| IBIS file stm32f413_f423_wlcsp100.ibs
[IBIS ver] 4.2
[File name] stm32f413_f423_wlcsp100.ibs
[File Rev] 1.2
[Date]  18-05-2020
[Source] Data Created at STMicroelectronics
[Notes]  File originated from ELDO simulations. rev 1.1: removal of the rising/falling waveform I2C
[Disclaimer]  This information is for modeling purpose only and is
   not guaranted. The information is subject to change without
   notice.
[Copyright] Copyright 2020 STMicroelectronics Inc.
|   Component stm32f413_f423_wlcsp100
[Component] stm32f413_f423_wlcsp100
[Manufacturer] STMicroelectronics
[Package]
| variable   typ   min   max
R_pkg   0.0   0.0   0.0
L_pkg   0.0H   0.0H   0.0H
C_pkg   0.0F   0.0F   0.0F
[Pin]  signal_name   model_name   R_pin   L_pin   C_pin
1 PA14 io8p_arsudq_ft
A10 PE4 io8p_arsudq_ft
A2 PC12 io8p_arsudq_ft
A3 PD2 io8p_arsudq_ft
A4 PD5 io8p_arsudq_ft
A5 PD7 io8p_arsudq_ft
A6 PB5 io8p_ar3wsudq_ft
A7 PB8 io8p_arsudq_i2cin_ft
A8 VSS_3 GND
A9 VDD_3 POWER
B1 VDD_2_0 POWER
B10 VBAT POWER
B2 VSS_2_0 GND
B3 PC11 io8p_arsudq_ft
B4 PD1 io8p_arsudq_ft
B5 PD3 io8p_arsudq_ft
B6 PD6 io8p_arsudq_ft
B7 PB6 io8p_arsudq_i2cin_ft
B8 PE0 io8p_arsudq_ft
B9 PE2 io8p_arsudq_ft
C1 VCAP2_0 POWER
C10 PC13-ANTI_TAMP io8p_arwsudq_ft_v33
C2 PA15 io8p_arsudq_ft
C3 PA13 io8p_arsudq_ft
C4 PA10 io8usb_id_otg_ft
C5 PD0 io8p_arsudq_ft
C6 PD4 io8p_arsudq_ft
C7 PB4 io8p_arsudq_i2cin_ft
C8 PE1 io8p_arsudq_ft
C9 PE3 io8p_arsudq_ft
D1 PA11 io8usb_lsfs_otg_ft
D10 PC14-OSC32_IN io8p_arwsudq_ft
D2 PA12 io8usb_lsfs_otg_ft
D3 PA9 io8usb_vbus_otg_ft
D4 PA8 io8p_arsudq_i2cin_ft
D5 PD14 io8p_arsudq_i2c_ft
D6 PB3 io8p_arsudq_i2c_ft
D7 PB7 io8p_arsudq_i2cin_ft
D8 VSS GND
D9 PE5 io8p_arsudq_ft
E1 PC9 io8p_arsudq_i2cin_ft
E10 VSS_5 GND
E2 PC8 io8p_arsudq_ft
E3 PC7 io8p_arsudq_i2c_ft
E4 PB12 io8p_arsudq_ft
E5 PA4 io8p_ar3wsudq_ft
E6 BOOT0 vpp_test_hv
E7 PB9 io8p_arsudq_i2cin_ft
E8 PE6 io8p_arsudq_ft
E9 PC15-OSC32_OUT io8p_arsudq_ft
F1 PC6 io8p_arsudq_i2c_ft
F10 VDD_5 POWER
F2 VDD_2_USB33 POWER
F3 PD10 io8p_arsudq_ft
F4 PE11 io8p_arsudq_ft
F5 PA5 io8p_ar3wsudq_ft
F6 PC3 io8p_arwsudq_ft
F7 PC0 io8p_arwsudq_ft_v33
F8 NRST ioreset_ft_v33
F9 PH0-OSC_IN io8p_arsudq_ft
G1 PD15 io8p_arsudq_i2c_ft
G10 PH1-OSC_OUT io8p_arsudq_ft
G2 PD13 io8p_arsudq_i2c_ft
G3 PD9 io8p_arsudq_ft
G4 PE15 io8p_ar3wsudq_ft
G5 PB2 io8p_arwsudq_ft
G6 PC5 io8p_arwsudq_ft
G7 PA3 io8p_arwsudq_ft
G8 VDDA POWER
G9 PC2 io8p_arwsudq_ft
H1 PD12 io8p_arsudq_i2c_ft
H10 PC1 io8p_arwsudq_ft_v33
H2 PB13 io8p_arsudq_ft
H3 PB10 io8p_arsudq_i2c_ft
H4 PE13 io8p_arsudq_ft
H5 PE7 io8p_arsudq_ft
H6 PC4 io8p_arwsudq_ft
H7 VSS_4 GND
H8 PA0-WKUP io8p_arwsudq_ft_v33
H9 VSSA GND
J1 PD11 io8p_arsudq_ft
J10 VREF+ POWER
J2 PB14 io8p_arsudq_i2c_ft
J3 VCAP1_0 POWER
J4 PE12 io8p_arsudq_ft
J5 PE9 io8p_arsudq_ft
J6 PB1 io8p_ar3wsudq_ft
J7 PA7 io8p_arwsudq_ft
J8 VDD_4 POWER
J9 PA2 io8p_arwsudq_ft
K1 PB15 io8p_arsudq_i2c_ft
K10 PA1 io8p_arwsudq_ft
K2 VDD_1_0 POWER
K3 VSS_1_0 GND
K4 PE14 io8p_arsudq_ft
K5 PE10 io8p_arsudq_ft
K6 PE8 io8p_arsudq_ft
K7 PB0 io8p_ar3wsudq_ft
K8 PA6 io8p_ar3wsudq_ft
K9 BYPASS_USER GND
[Model Selector] io8p_ar3wsudq_ft
io8p00_ar3wsudq_ft_pd_lv  "SPEED00 1P8V, PD=40kOhm"
io8p00_ar3wsudq_ft_pu_lv  "SPEED00 1P8V, PU=40kOhm"
io8p00_ar3wsudq_ft_lv  "SPEED00 1P8V"
io8p01_ar3wsudq_ft_pd_lv  "SPEED01 1P8V, PD=40kOhm"
io8p01_ar3wsudq_ft_pu_lv  "SPEED01 1P8V, PU=40kOhm"
io8p01_ar3wsudq_ft_lv  "SPEED01 1P8V"
io8p10_ar3wsudq_ft_pd_lv  "SPEED10 1P8V, PD=40kOhm"
io8p10_ar3wsudq_ft_pu_lv  "SPEED10 1P8V, PU=40kOhm"
io8p10_ar3wsudq_ft_lv  "SPEED10 1P8V"
io8p11_ar3wsudq_ft_pd_lv  "SPEED11 1P8V, PD=40kOhm"
io8p11_ar3wsudq_ft_pu_lv  "SPEED11 1P8V, PU=40kOhm"
io8p11_ar3wsudq_ft_lv  "SPEED11 1P8V"
io8p00_ar3wsudq_ft_pd  "SPEED00, PD=40kOhm"
io8p00_ar3wsudq_ft_pu  "SPEED00, PU=40kOhm"
io8p00_ar3wsudq_ft  "SPEED00"
io8p01_ar3wsudq_ft_pd  "SPEED01, PD=40kOhm"
io8p01_ar3wsudq_ft_pu  "SPEED01, PU=40kOhm"
io8p01_ar3wsudq_ft  "SPEED01"
io8p10_ar3wsudq_ft_pd  "SPEED10, PD=40kOhm"
io8p10_ar3wsudq_ft_pu  "SPEED10, PU=40kOhm"
io8p10_ar3wsudq_ft  "SPEED10"
io8p11_ar3wsudq_ft_pd  "SPEED11, PD=40kOhm"
io8p11_ar3wsudq_ft_pu  "SPEED11, PU=40kOhm"
io8p11_ar3wsudq_ft  "SPEED11"
[Model Selector] io8p_arsudq_ft
io8p00_arsudq_ft_pd_lv  "SPEED00 1P8V, PD=40kOhm"
io8p00_arsudq_ft_pu_lv  "SPEED00 1P8V, PU=40kOhm"
io8p00_arsudq_ft_lv  "SPEED00 1P8V"
io8p01_arsudq_ft_pd_lv  "SPEED01 1P8V, PD=40kOhm"
io8p01_arsudq_ft_pu_lv  "SPEED01 1P8V, PU=40kOhm"
io8p01_arsudq_ft_lv  "SPEED01 1P8V"
io8p10_arsudq_ft_pd_lv  "SPEED10 1P8V, PD=40kOhm"
io8p10_arsudq_ft_pu_lv  "SPEED10 1P8V, PU=40kOhm"
io8p10_arsudq_ft_lv  "SPEED10 1P8V"
io8p11_arsudq_ft_pd_lv  "SPEED11 1P8V, PD=40kOhm"
io8p11_arsudq_ft_pu_lv  "SPEED11 1P8V, PU=40kOhm"
io8p11_arsudq_ft_lv  "SPEED11 1P8V"
io8p00_arsudq_ft_pd  "SPEED00, PD=40kOhm"
io8p00_arsudq_ft_pu  "SPEED00, PU=40kOhm"
io8p00_arsudq_ft  "SPEED00"
io8p01_arsudq_ft_pd  "SPEED01, PD=40kOhm"
io8p01_arsudq_ft_pu  "SPEED01, PU=40kOhm"
io8p01_arsudq_ft  "SPEED01"
io8p10_arsudq_ft_pd  "SPEED10, PD=40kOhm"
io8p10_arsudq_ft_pu  "SPEED10, PU=40kOhm"
io8p10_arsudq_ft  "SPEED10"
io8p11_arsudq_ft_pd  "SPEED11, PD=40kOhm"
io8p11_arsudq_ft_pu  "SPEED11, PU=40kOhm"
io8p11_arsudq_ft  "SPEED11"
[Model Selector] io8p_arsudq_i2c_ft
io8prog_1v8_i2c_pd  "5V Tol GPIO 1.8V range i2c functionality with pull down"
io8prog_1v8_i2c_pu  "5V Tol GPIO 1.8V range i2c functionality with pull up"
io8prog_1v8_i2c  "5V Tol GPIO 1.8V range i2c functionality"
io8prog_3v3_i2c_pd  "5V Tol GPIO 3.3V range i2c functionality with pull down"
io8prog_3v3_i2c_pu  "5V Tol GPIO 3.3V range i2c functionality with pull up"
io8prog_3v3_i2c  "5V Tol GPIO 3.3V range i2c functionality"
io8prog_1v8_pd_00  "5V Tol GPIO 1.8V range with pd speed 00"
io8prog_1v8_pu_00  "5V Tol GPIO 1.8V range with pu speed 00"
io8prog_1v8_00  "5V Tol GPIO 1.8V range speed 00"
io8prog_3v3_pd_00  "5V Tol GPIO 3.3V range with pd speed 00"
io8prog_3v3_pu_00  "5V Tol GPIO 3.3V range with pu speed 00"
io8prog_3v3_00  "5V Tol GPIO 3.3V range speed 00"
io8prog_1v8_pd_01  "5V Tol GPIO 1.8V range with pd speed 01"
io8prog_1v8_pu_01  "5V Tol GPIO 1.8V range with pu speed 01"
io8prog_1v8_01  "5V Tol GPIO 1.8V range speed 01"
io8prog_3v3_pd_01  "5V Tol GPIO 3.3V range with pd speed 01"
io8prog_3v3_pu_01  "5V Tol GPIO 3.3V range with pu speed 01"
io8prog_3v3_01  "5V Tol GPIO 3.3V range speed 01"
io8prog_1v8_pd_10  "5V Tol GPIO 1.8V range with pd speed 10"
io8prog_1v8_pu_10  "5V Tol GPIO 1.8V range with pu speed 10"
io8prog_1v8_10  "5V Tol GPIO 1.8V range speed 10"
io8prog_3v3_pd_10  "5V Tol GPIO 3.3V range with pd speed 10"
io8prog_3v3_pu_10  "5V Tol GPIO 3.3V range with pu speed 10"
io8prog_3v3_10  "5V Tol GPIO 3.3V range speed 10"
io8prog_1v8_pd_11  "5V Tol GPIO 1.8V range with pd speed 11"
io8prog_1v8_pu_11  "5V Tol GPIO 1.8V range with pu speed 11"
io8prog_1v8_11  "5V Tol GPIO 1.8V range speed 11"
io8prog_3v3_pd_11  "5V Tol GPIO 3.3V range with pd speed 11"
io8prog_3v3_pu_11  "5V Tol GPIO 3.3V range with pu speed 11"
io8prog_3v3_11  "5V Tol GPIO 3.3V range speed 11"
[Model Selector] io8p_arsudq_i2cin_ft
io8p00_arsudq_i2cin_ft_pd_lv  "SPEED00 1P8V, PD=40kOhm"
io8p00_arsudq_i2cin_ft_pu_lv  "SPEED00 1P8V, PU=40kOhm"
io8p00_arsudq_i2cin_ft_lv  "SPEED00 1P8V"
io8p01_arsudq_i2cin_ft_pd_lv  "SPEED01 1P8V, PD=40kOhm"
io8p01_arsudq_i2cin_ft_pu_lv  "SPEED01 1P8V, PU=40kOhm"
io8p01_arsudq_i2cin_ft_lv  "SPEED01 1P8V"
io8p10_arsudq_i2cin_ft_pd_lv  "SPEED10 1P8V, PD=40kOhm"
io8p10_arsudq_i2cin_ft_pu_lv  "SPEED10 1P8V, PU=40kOhm"
io8p10_arsudq_i2cin_ft_lv  "SPEED10 1P8V"
io8p11_arsudq_i2cin_ft_pd_lv  "SPEED11 1P8V, PD=40kOhm"
io8p11_arsudq_i2cin_ft_pu_lv  "SPEED11 1P8V, PU=40kOhm"
io8p11_arsudq_i2cin_ft_lv  "SPEED11 1P8V"
io8p00_arsudq_i2cin_ft_pd  "SPEED00, PD=40kOhm"
io8p00_arsudq_i2cin_ft_pu  "SPEED00, PU=40kOhm"
io8p00_arsudq_i2cin_ft  "SPEED00"
io8p01_arsudq_i2cin_ft_pd  "SPEED01, PD=40kOhm"
io8p01_arsudq_i2cin_ft_pu  "SPEED01, PU=40kOhm"
io8p01_arsudq_i2cin_ft  "SPEED01"
io8p10_arsudq_i2cin_ft_pd  "SPEED10, PD=40kOhm"
io8p10_arsudq_i2cin_ft_pu  "SPEED10, PU=40kOhm"
io8p10_arsudq_i2cin_ft  "SPEED10"
io8p11_arsudq_i2cin_ft_pd  "SPEED11, PD=40kOhm"
io8p11_arsudq_i2cin_ft_pu  "SPEED11, PU=40kOhm"
io8p11_arsudq_i2cin_ft  "SPEED11"
[Model Selector] io8p_arwsudq_ft
io8p00_arwsudq_ft_pd_lv  "SPEED00 1P8V, PD=40kOhm"
io8p00_arwsudq_ft_pu_lv  "SPEED00 1P8V, PU=40kOhm"
io8p00_arwsudq_ft_lv  "SPEED00 1P8V"
io8p01_arwsudq_ft_pd_lv  "SPEED01 1P8V, PD=40kOhm"
io8p01_arwsudq_ft_pu_lv  "SPEED01 1P8V, PU=40kOhm"
io8p01_arwsudq_ft_lv  "SPEED01 1P8V"
io8p10_arwsudq_ft_pd_lv  "SPEED10 1P8V, PD=40kOhm"
io8p10_arwsudq_ft_pu_lv  "SPEED10 1P8V, PU=40kOhm"
io8p10_arwsudq_ft_lv  "SPEED10 1P8V"
io8p11_arwsudq_ft_pd_lv  "SPEED11 1P8V, PD=40kOhm"
io8p11_arwsudq_ft_pu_lv  "SPEED11 1P8V, PU=40kOhm"
io8p11_arwsudq_ft_lv  "SPEED11 1P8V"
io8p00_arwsudq_ft_pd  "SPEED00, PD=40kOhm"
io8p00_arwsudq_ft_pu  "SPEED00, PU=40kOhm"
io8p00_arwsudq_ft  "SPEED00"
io8p01_arwsudq_ft_pd  "SPEED01, PD=40kOhm"
io8p01_arwsudq_ft_pu  "SPEED01, PU=40kOhm"
io8p01_arwsudq_ft  "SPEED01"
io8p10_arwsudq_ft_pd  "SPEED10, PD=40kOhm"
io8p10_arwsudq_ft_pu  "SPEED10, PU=40kOhm"
io8p10_arwsudq_ft  "SPEED10"
io8p11_arwsudq_ft_pd  "SPEED11, PD=40kOhm"
io8p11_arwsudq_ft_pu  "SPEED11, PU=40kOhm"
io8p11_arwsudq_ft  "SPEED11"
[Model Selector] io8p_arwsudq_ft_v33
io8p00_arwsudq_ft_v33_pd_lv  "SPEED00 1P8V, PD=40kOhm"
io8p00_arwsudq_ft_v33_pu_lv  "SPEED00 1P8V, PU=40kOhm"
io8p00_arwsudq_ft_v33_lv  "SPEED00 1P8V"
io8p01_arwsudq_ft_v33_pd_lv  "SPEED01 1P8V, PD=40kOhm"
io8p01_arwsudq_ft_v33_pu_lv  "SPEED01 1P8V, PU=40kOhm"
io8p01_arwsudq_ft_v33_lv  "SPEED01 1P8V"
io8p10_arwsudq_ft_v33_pd_lv  "SPEED10 1P8V, PD=40kOhm"
io8p10_arwsudq_ft_v33_pu_lv  "SPEED10 1P8V, PU=40kOhm"
io8p10_arwsudq_ft_v33_lv  "SPEED10 1P8V"
io8p11_arwsudq_ft_v33_pd_lv  "SPEED11 1P8V, PD=40kOhm"
io8p11_arwsudq_ft_v33_pu_lv  "SPEED11 1P8V, PU=40kOhm"
io8p11_arwsudq_ft_v33_lv  "SPEED11 1P8V"
io8p00_arwsudq_ft_v33_pd  "SPEED00, PD=40kOhm"
io8p00_arwsudq_ft_v33_pu  "SPEED00, PU=40kOhm"
io8p00_arwsudq_ft_v33  "SPEED00"
io8p01_arwsudq_ft_v33_pd  "SPEED01, PD=40kOhm"
io8p01_arwsudq_ft_v33_pu  "SPEED01, PU=40kOhm"
io8p01_arwsudq_ft_v33  "SPEED01"
io8p10_arwsudq_ft_v33_pd  "SPEED10, PD=40kOhm"
io8p10_arwsudq_ft_v33_pu  "SPEED10, PU=40kOhm"
io8p10_arwsudq_ft_v33  "SPEED10"
io8p11_arwsudq_ft_v33_pd  "SPEED11, PD=40kOhm"
io8p11_arwsudq_ft_v33_pu  "SPEED11, PU=40kOhm"
io8p11_arwsudq_ft_v33  "SPEED11"
[Model Selector] io8usb_id_otg_ft
io8p00_id_otg_ft_pd_lv  "SPEED00 1P8V, PD=14kOhm"
io8p00_id_otg_ft_pu_lv  "SPEED00 1P8V, PU=14kOhm"
io8p00_id_otg_ft_lv  "SPEED00 1P8V"
io8p01_id_otg_ft_pd_lv  "SPEED01 1P8V, PD=14kOhm"
io8p01_id_otg_ft_pu_lv  "SPEED01 1P8V, PU=14kOhm"
io8p01_id_otg_ft_lv  "SPEED01 1P8V"
io8p10_id_otg_ft_pd_lv  "SPEED10 1P8V, PD=14kOhm"
io8p10_id_otg_ft_pu_lv  "SPEED10 1P8V, PU=14kOhm"
io8p10_id_otg_ft_lv  "SPEED10 1P8V"
io8p11_id_otg_ft_pd_lv  "SPEED11 1P8V, PD=14kOhm"
io8p11_id_otg_ft_pu_lv  "SPEED11 1P8V, PU=14kOhm"
io8p11_id_otg_ft_lv  "SPEED11 1P8V"
io8p00_id_otg_ft_pd  "SPEED00, PD=14kOhm"
io8p00_id_otg_ft_pu  "SPEED00, PU=14kOhm"
io8p00_id_otg_ft  "SPEED00"
io8p01_id_otg_ft_pd  "SPEED01, PD=14kOhm"
io8p01_id_otg_ft_pu  "SPEED01, PU=14kOhm"
io8p01_id_otg_ft  "SPEED01"
io8p10_id_otg_ft_pd  "SPEED10, PD=14kOhm"
io8p10_id_otg_ft_pu  "SPEED10, PU=14kOhm"
io8p10_id_otg_ft  "SPEED10"
io8p11_id_otg_ft_pd  "SPEED11, PD=14kOhm"
io8p11_id_otg_ft_pu  "SPEED11, PU=14kOhm"
io8p11_id_otg_ft  "SPEED11"
[Model Selector] io8usb_lsfs_otg_ft
io8usb_ls_otg_ft_dpdn_pd  "LS USB DP/DN IO + PD=20kOhm"
io8usb_ls_otg_ft_dpdn_pupu2  "LS USB DP/DN IO + PU/PU2=2.2kOhm"
io8usb_ls_otg_ft_dpdn_pu2  "LS USB DP/DN IO + PU2=1.2kOhm"
io8usb_ls_otg_ft_dpdn_pu  "LS USB DP/DN IO + PU=1.2kOhm"
io8usb_ls_otg_ft_dpdn  "LS USB DP/DN IO"
io8usb_fs_otg_ft_dpdn_pd  "HS USB DP/DN IO + PD=20kOhm"
io8usb_fs_otg_ft_dpdn_pupu2  "HS USB DP/DN IO + PU/PU2=2.2kOhm"
io8usb_fs_otg_ft_dpdn_pu2  "HS USB DP/DN IO + PU2=1.2kOhm"
io8usb_fs_otg_ft_dpdn_pu  "HS USB DP/DN IO + PU=1.2kOhm"
io8usb_fs_otg_ft_dpdn  "HS USB DP/DN IO"
io8p00_lsfs_otg_ft_pd_lv  "SPEED00 1P8V, PD=40kOhm"
io8p00_lsfs_otg_ft_pu_lv  "SPEED00 1P8V, PU=40kOhm"
io8p00_lsfs_otg_ft_lv  "SPEED00 1P8V"
io8p01_lsfs_otg_ft_pd_lv  "SPEED01 1P8V, PD=40kOhm"
io8p01_lsfs_otg_ft_pu_lv  "SPEED01 1P8V, PU=40kOhm"
io8p01_lsfs_otg_ft_lv  "SPEED01 1P8V"
io8p10_lsfs_otg_ft_pd_lv  "SPEED10 1P8V, PD=40kOhm"
io8p10_lsfs_otg_ft_pu_lv  "SPEED10 1P8V, PU=40kOhm"
io8p10_lsfs_otg_ft_lv  "SPEED10 1P8V"
io8p11_lsfs_otg_ft_pd_lv  "SPEED11 1P8V, PD=40kOhm"
io8p11_lsfs_otg_ft_pu_lv  "SPEED11 1P8V, PU=40kOhm"
io8p11_lsfs_otg_ft_lv  "SPEED11 1P8V"
io8p00_lsfs_otg_ft_pd  "SPEED00, PD=40kOhm"
io8p00_lsfs_otg_ft_pu  "SPEED00, PU=40kOhm"
io8p00_lsfs_otg_ft  "SPEED00"
io8p01_lsfs_otg_ft_pd  "SPEED01, PD=40kOhm"
io8p01_lsfs_otg_ft_pu  "SPEED01, PU=40kOhm"
io8p01_lsfs_otg_ft  "SPEED01"
io8p10_lsfs_otg_ft_pd  "SPEED10, PD=40kOhm"
io8p10_lsfs_otg_ft_pu  "SPEED10, PU=40kOhm"
io8p10_lsfs_otg_ft  "SPEED10"
io8p11_lsfs_otg_ft_pd  "SPEED11, PD=40kOhm"
io8p11_lsfs_otg_ft_pu  "SPEED11, PU=40kOhm"
io8p11_lsfs_otg_ft  "SPEED11"
[Model Selector] io8usb_vbus_otg_ft
io8psenb_vbus_otg_ft  "VBUS PULSE, SENSE VB"
io8psenab_vbus_otg_ft  "VBUS PULSE, SENSE VA and VB"
io8psena_vbus_otg_ft  "VBUS PULSE, SENSE VA"
io8psen_vbus_otg_ft  "VBUS PULSE"
io8p00_vbus_otg_ft_pd_lv  "SPEED00 1P8V, PD=40kOhm"
io8p00_vbus_otg_ft_pu_lv  "SPEED00 1P8V, PU=40kOhm"
io8p00_vbus_otg_ft_lv  "SPEED00 1P8V"
io8p01_vbus_otg_ft_pd_lv  "SPEED01 1P8V, PD=40kOhm"
io8p01_vbus_otg_ft_pu_lv  "SPEED01 1P8V, PU=40kOhm"
io8p01_vbus_otg_ft_lv  "SPEED01 1P8V"
io8p10_vbus_otg_ft_pd_lv  "SPEED10 1P8V, PD=40kOhm"
io8p10_vbus_otg_ft_pu_lv  "SPEED10 1P8V, PU=40kOhm"
io8p10_vbus_otg_ft_lv  "SPEED10 1P8V"
io8p11_vbus_otg_ft_pd_lv  "SPEED11 1P8V, PD=40kOhm"
io8p11_vbus_otg_ft_pu_lv  "SPEED11 1P8V, PU=40kOhm"
io8p11_vbus_otg_ft_lv  "SPEED11 1P8V"
io8p00_vbus_otg_ft_pd  "SPEED00, PD=40kOhm"
io8p00_vbus_otg_ft_pu  "SPEED00, PU=40kOhm"
io8p00_vbus_otg_ft  "SPEED00"
io8p01_vbus_otg_ft_pd  "SPEED01, PD=40kOhm"
io8p01_vbus_otg_ft_pu  "SPEED01, PU=40kOhm"
io8p01_vbus_otg_ft  "SPEED01"
io8p10_vbus_otg_ft_pd  "SPEED10, PD=40kOhm"
io8p10_vbus_otg_ft_pu  "SPEED10, PU=40kOhm"
io8p10_vbus_otg_ft  "SPEED10"
io8p11_vbus_otg_ft_pd  "SPEED11, PD=40kOhm"
io8p11_vbus_otg_ft_pu  "SPEED11, PU=40kOhm"
io8p11_vbus_otg_ft  "SPEED11"
[Model Selector] ioreset_ft_v33
ioreset_ft_v33_pu_lv  "IORESET 1P8V + PU=40kOhm"
ioreset_ft_v33_nopu_lv  "IORESET 1P8V"
ioreset_ft_v33_pu  "IORESET + PU=40kOhm"
ioreset_ft_v33_nopu  "IORESET"
[Model Selector] vpp_test_hv
vpp_test_hv_2p4  "Input Buffer 1P8V"
vpp_test_hv_3p3  "Input Buffer"
| Models and submodels in the file (242): io8p00_ar3wsudq_ft_pd_lv (I/O), io8p00_ar3wsudq_ft_pu_lv (I/O), io8p00_ar3wsudq_ft_lv (I/O), io8p01_ar3wsudq_ft_pd_lv (I/O), io8p01_ar3wsudq_ft_pu_lv (I/O), io8p01_ar3wsudq_ft_lv (I/O), io8p10_ar3wsudq_ft_pd_lv (I/O), io8p10_ar3wsudq_ft_pu_lv (I/O), io8p10_ar3wsudq_ft_lv (I/O), io8p11_ar3wsudq_ft_pd_lv (I/O), io8p11_ar3wsudq_ft_pu_lv (I/O), io8p11_ar3wsudq_ft_lv (I/O), io8p00_ar3wsudq_ft_pd (I/O), io8p00_ar3wsudq_ft_pu (I/O), io8p00_ar3wsudq_ft (I/O), io8p01_ar3wsudq_ft_pd (I/O), io8p01_ar3wsudq_ft_pu (I/O), io8p01_ar3wsudq_ft (I/O), io8p10_ar3wsudq_ft_pd (I/O), io8p10_ar3wsudq_ft_pu (I/O), io8p10_ar3wsudq_ft (I/O), io8p11_ar3wsudq_ft_pd (I/O), io8p11_ar3wsudq_ft_pu (I/O), io8p11_ar3wsudq_ft (I/O), io8p00_arsudq_ft_pd_lv (I/O), io8p00_arsudq_ft_pu_lv (I/O), io8p00_arsudq_ft_lv (I/O), io8p01_arsudq_ft_pd_lv (I/O), io8p01_arsudq_ft_pu_lv (I/O), io8p01_arsudq_ft_lv (I/O), io8p10_arsudq_ft_pd_lv (I/O), io8p10_arsudq_ft_pu_lv (I/O), io8p10_arsudq_ft_lv (I/O), io8p11_arsudq_ft_pd_lv (I/O), io8p11_arsudq_ft_pu_lv (I/O), io8p11_arsudq_ft_lv (I/O), io8p00_arsudq_ft_pd (I/O), io8p00_arsudq_ft_pu (I/O), io8p00_arsudq_ft (I/O), io8p01_arsudq_ft_pd (I/O), io8p01_arsudq_ft_pu (I/O), io8p01_arsudq_ft (I/O), io8p10_arsudq_ft_pd (I/O), io8p10_arsudq_ft_pu (I/O), io8p10_arsudq_ft (I/O), io8p11_arsudq_ft_pd (I/O), io8p11_arsudq_ft_pu (I/O), io8p11_arsudq_ft (I/O), io8prog_1v8_i2c_pd (I/O), io8prog_1v8_i2c_pu (I/O), io8prog_1v8_i2c (I/O), io8prog_3v3_i2c_pd (I/O), io8prog_3v3_i2c_pu (I/O), io8prog_3v3_i2c (I/O), io8prog_1v8_pd_00 (I/O), io8prog_1v8_pu_00 (I/O), io8prog_1v8_00 (I/O), io8prog_3v3_pd_00 (I/O), io8prog_3v3_pu_00 (I/O), io8prog_3v3_00 (I/O), io8prog_1v8_pd_01 (I/O), io8prog_1v8_pu_01 (I/O), io8prog_1v8_01 (I/O), io8prog_3v3_pd_01 (I/O), io8prog_3v3_pu_01 (I/O), io8prog_3v3_01 (I/O), io8prog_1v8_pd_10 (I/O), io8prog_1v8_pu_10 (I/O), io8prog_1v8_10 (I/O), io8prog_3v3_pd_10 (I/O), io8prog_3v3_pu_10 (I/O), io8prog_3v3_10 (I/O), io8prog_1v8_pd_11 (I/O), io8prog_1v8_pu_11 (I/O), io8prog_1v8_11 (I/O), io8prog_3v3_pd_11 (I/O), io8prog_3v3_pu_11 (I/O), io8prog_3v3_11 (I/O), io8p00_arsudq_i2cin_ft_pd_lv (I/O), io8p00_arsudq_i2cin_ft_pu_lv (I/O)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
